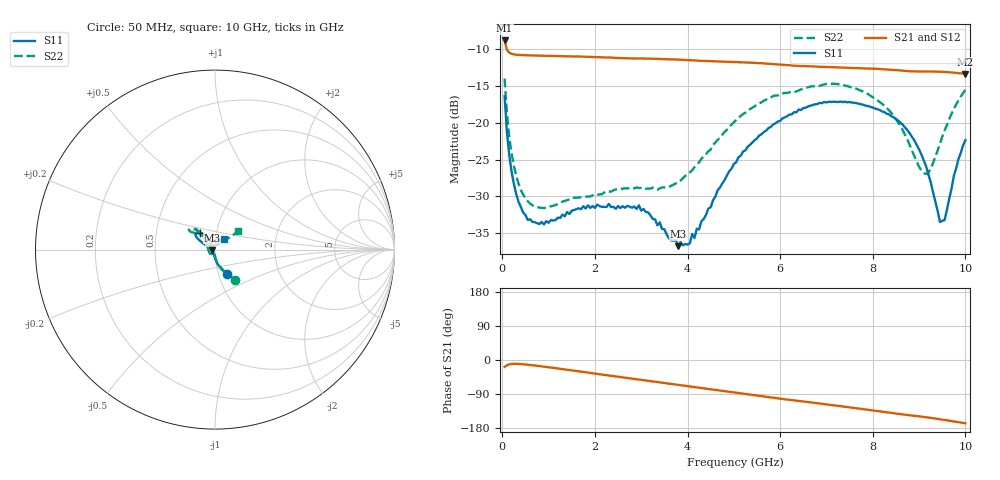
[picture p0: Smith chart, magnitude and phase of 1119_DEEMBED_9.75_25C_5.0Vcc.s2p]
!Hittite Microwave Corp.
!Digital Attenuator/PhaseShifter Rev 1.4.0
!Filename: C:\DATA\DATA\1119_DEEMBED_9.75_25C_5.0Vcc.s2p
!VNA ID: Agilent Technologies,N5224A,MY51441122,A.10.45.03
!Device type:
!2 Port Calibration.
!Temp(C): 25
!Lot Number:
!Serial Number:
!Operator:
!Misc:
!Attenuator:  9.750
# GHZ S DB R 50.0
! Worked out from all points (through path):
!   200 points, 50 MHz to 10 GHz, reference 50 ohm
!   highest |S21| = -8.82 dB at 50 MHz (marker M1); lowest = -13.4 dB at 10 GHz (marker M2)
!   group delay of S21, straight-line fit = 44.8 ps
!   lowest |S11| = -36.8 dB at 3.8 GHz (marker M3), VSWR 1.03, Z = 48.6 - j0.244 ohm
!   |S11| at or under -10 dB: start of sweep to end of sweep
!   |S22| runs from -31.6 to -14.0 dB; largest |S21 - S12| = 0.00094
!   S11 on the Smith chart (normalised r, x): 50 MHz: 1.10, -0.31; 6.5 GHz: 0.83, +0.16; 10 GHz: 1.09, +0.13
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0.05  -16.39 -63.7  -8.82 -18.0  -8.81 -18.0  -14.00 -56.8
0.1  -21.29 -78.7  -10.09 -13.9  -10.09 -13.9  -18.75 -72.1
0.2  -26.65 -91.2  -10.63 -10.5  -10.63 -10.5  -24.15 -82.7
0.35  -30.74 -100.4  -10.78 -10.3  -10.79 -10.3  -28.27 -87.6
0.55  -33.20 -110.2  -10.84 -12.4  -10.84 -12.4  -30.67 -92.9
0.9  -33.82 -118.0  -10.90 -17.6  -10.90 -17.6  -31.58 -96.5
1.75  -31.34 -126.8  -11.02 -31.5  -11.02 -31.6  -30.03 -110.7
2.95  -31.22 -126.3  -11.27 -51.3  -11.28 -51.4  -28.87 -148.2
3.4  -33.53 -141.9  -11.33 -59.0  -11.33 -59.0  -28.91 -168.7
3.8  -36.77 -170.0  -11.42 -65.9  -11.43 -65.9  -28.14 170.0
4.15  -35.66 149.8  -11.53 -71.7  -11.55 -71.8  -26.03 151.4
5.05  -25.36 123.1  -11.75 -86.2  -11.77 -86.3  -19.64 130.0
6.5  -18.01 131.6  -12.30 -109.4  -12.31 -109.4  -15.36 138.6
6.7  -17.60 133.7  -12.34 -112.5  -12.35 -112.5  -15.06 140.0
7.65  -17.34 143.2  -12.58 -127.3  -12.59 -127.3  -15.39 144.0
8.35  -18.87 147.6  -12.77 -138.8  -12.78 -138.8  -18.30 134.8
8.75  -21.02 150.7  -12.99 -145.1  -12.99 -145.1  -22.33 121.4
9.1  -25.10 152.9  -13.04 -150.2  -13.05 -150.2  -26.84 91.3
9.45  -33.48 116.9  -13.06 -156.3  -13.07 -156.3  -22.87 47.6
9.55  -33.22 84.1  -13.09 -158.2  -13.10 -158.2  -21.06 42.6
9.75  -27.24 53.4  -13.19 -162.1  -13.21 -162.1  -18.13 38.7
10  -22.37 50.6  -13.37 -167.1  -13.37 -167.0  -15.51 39.3
